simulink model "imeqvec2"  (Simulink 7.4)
settings: Solver=ode45  StartTime=0.0  StopTime=1  MaxStep=1e-3  RelTol=1e-3
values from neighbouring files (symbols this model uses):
  H = 0.60    (= 0.6)    [IMabc2.m]    (also in IMcur0.m = 0.3; imdef0vec.m = 0.3; imdef1vec.m = 0.3; imdef2vec.m = 0.3)
  ic = [fs0 fr0]    [imdef0vec.m]    (also in imdef1vec.m; imdef2vec.m = F; imic2.m = [phids phiqs phidr phiqr n0]'; imic3.m = [phids phiqs phidr phiqr n0]')
  Lm = eval(get(hLm,'String'))    [im3d.m]    (also in IMabc2.m = 4.5; imabcparam.m = 0.0847; IMabcrun0.m = 0.0847; IMabcrun1.m = 0.0847)
  Lrl = eval(get(hLr,'String'))    [im3d.m]    (also in IMabc2.m = 0.1; imabcparam.m = 0.0025; IMabcrun0.m = 0.0025; IMabcrun1.m = 0.0025)
  Lsl = eval(get(hLs,'String'))    [im3d.m]    (also in IMabc2.m = 0.1; imabcparam.m = 0.0025; IMabcrun0.m = 0.0025; IMabcrun1.m = 0.0025)
  n0 = 0.98    [imdef0vec.m]    (also in imdef1vec.m = 0.978; imdef2vec.m; imdefrotflux.m; imdefSIvec1.m = 0.95)
  Rr = input('Rotor resistance)[default = 2] =')    [Actac.m]    (also in im1phase.m = 0.3; im3d.m = eval(get(hRr,'String')); IMabc2.m = 0.02; imabcparam.m = 0.408)
  Rs = eval(get(hRs,'String'))    [im3d.m]    (also in IMabc2.m = 0.01; imabcparam.m = 0.531; IMabcrun0.m = 0.531; IMabcrun1.m = 0.531)
  Tl0 = Is*conj(Is)*Req    [imdef0vec.m]    (also in imdef1vec.m; imdef2vec.m = Lm*(I(2)*I(3)-I(1)*I(4)); imdefrotflux.m; imdefSIvec1.m = Te0/To)
  vs = 1.0    (= 1)    [imdef0vec.m]    (also in imdef1vec.m; imdef2vec.m; imdefrotflux.m; imdefSIvec1.m)
  wk = ws    (= 1)    [imdef0vec.m]    (also in imdef1vec.m; imdef2vec.m; imdefrotflux.m; imdefSIvec1.m)
  wo = 2*pi*freq0    [calc0.m]    (also in IMabc2.m = 376.991118431; imabcparam.m = 376.991118431; IMabcrun0.m = 376.991118431; IMabcrun1.m = 376.991118431)

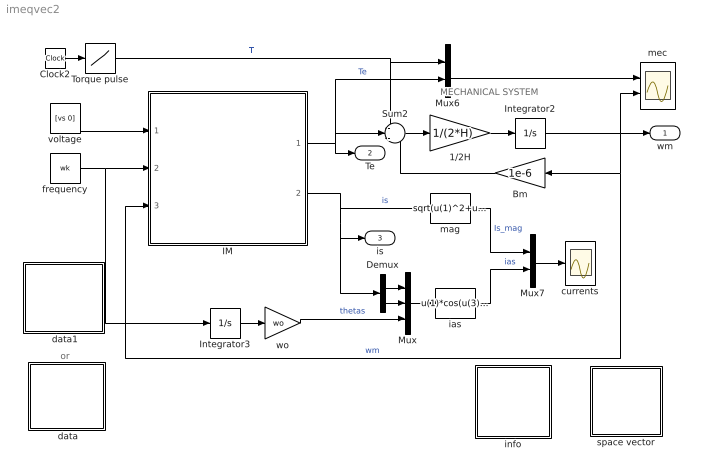
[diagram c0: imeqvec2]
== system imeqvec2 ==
  note: or
  note: MECHANICAL SYSTEM
  " data" : Subsystem
  " data1" : Subsystem
  1/2H : Gain  Gain=1/(2*H)  ParameterDataType=sfix(16)  ParameterScaling=2^0  OutDataType=sfix(16)  OutScaling=2^0
  Bm : Gain  Gain=1e-6  ParameterDataType=sfix(16)  ParameterScaling=2^0  OutDataType=sfix(16)  OutScaling=2^0
  Clock2 : Clock
  Demux : Demux  Outputs=2
  IM : Subsystem
  Integrator2 : Integrator  InitialCondition=n0
  Integrator3 : Integrator
  Mux : Mux  Inputs=3
  Mux6 : Mux  Inputs=2
  Mux7 : Mux  Inputs=2
  Sum2 : Sum  Inputs=-+-  OutDataType=sfix(16)  OutScaling=2^0
  Torque pulse : Lookup  InputValues=[0 0.1 0.1 0.5 0.5 2]  Table="[Tl0 Tl0  0 0 0.5 0.5]"  OutDataType=sfix(16)  OutScaling=2^0
  currents : Scope
  frequency : Constant  Value=wk  OutDataType=sfix(16)  OutScaling=2^0
  ias : Fcn  Expr=u(1)*cos(u(3))-u(2)*sin(u(3))
  info : Subsystem
  mag : Fcn  Expr=sqrt(u(1)^2+u(2)^2)
  mec : Scope  NumInputPorts=2
  space vector : Subsystem
  voltage : Constant  Value=[vs 0]  OutDataType=sfix(16)  OutScaling=2^0
  wo : Gain  Gain=wo  ParameterDataType=sfix(16)  ParameterScaling=2^0  OutDataType=sfix(16)  OutScaling=2^0
  wm : Outport
  Te : Outport  Port=2
  is : Outport  Port=3
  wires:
  voltage/1 -> IM/1(vs)
  frequency/1 -> Integrator3/1, IM/2(wk)
  Demux/1 -> Mux/1
  Demux/2 -> Mux/2
  Mux/1 -> ias/1
  ias/1 -> Mux7/2  "ias"
  mag/1 -> Mux7/1  "Is_mag"
  Mux7/1 -> currents/1
  IM/2(is) -> mag/1, Demux/1, is/1  "is"
  Sum2/1 -> 1/2H/1
  1/2H/1 -> Integrator2/1
  Mux6/1 -> mec/1
  IM/1(Te) -> Sum2/2, Mux6/2, Te/1  "Te"
  Bm/1 -> Sum2/3
  Integrator3/1 -> wo/1
  wo/1 -> Mux/3  "thetas"
  Integrator2/1 -> mec/2, wm/1, IM/3(wm), Bm/1  "wm"
  Clock2/1 -> Torque pulse/1
  Torque pulse/1 -> Mux6/1, Sum2/1  "Tl"

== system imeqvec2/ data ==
  note: This demo simulates the running of an induction motor in steady-state when a sudden input change is effected: a)torque step changes at constant voltage excitation b) voltage input sag at constant frequency and load torque c)simultaneous step changes in voltage magnitude and frequency
  note: Double click the block to enter the machine parameters and initial conditions and then run the simulation

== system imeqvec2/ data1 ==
  note: This demo simulates the running of an induction motor in steady-state when a sudden input change is effected: a)torque step changes at constant voltage excitation b) voltage input sag at constant frequency and load torque c)simultaneous step changes in voltage magnitude and frequency
  note: Double click the block to enter the machine parameters and initial conditions and then run the simulation

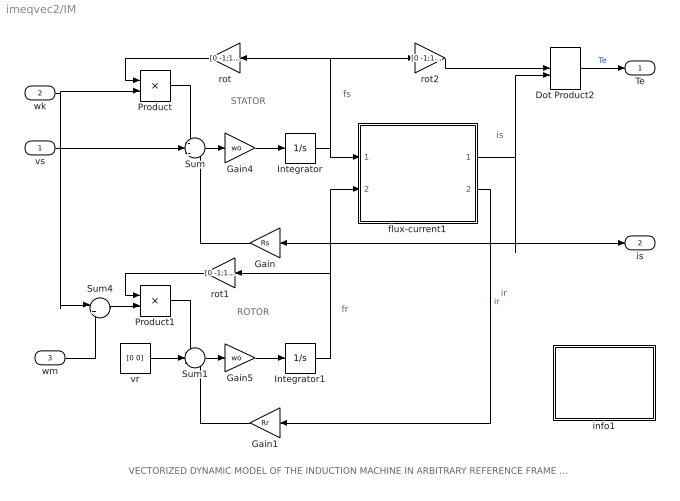
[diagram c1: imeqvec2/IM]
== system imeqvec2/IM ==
  note: ROTOR
  note: STATOR
  note: fs
  note: fr
  note: is
  note: VECTORIZED DYNAMIC MODEL OF THE INDUCTION MACHINE IN ARBITRARY REFERENCE FRAME (per unit formulation)
  note: ir
  vs : Inport  OutDataType=sfix(16)  OutScaling=2^0
  wk : Inport  Port=2  OutDataType=sfix(16)  OutScaling=2^0
  wm : Inport  Port=3  OutDataType=sfix(16)  OutScaling=2^0
  Dot Product2 : DotProduct  OutDataType=fixdt(1, 16)  OutScaling=2^-10
  Gain : Gain  Gain=Rs  ParameterDataType=sfix(16)  ParameterScaling=2^0  OutDataType=sfix(16)  OutScaling=2^0
  Gain1 : Gain  Gain=Rr  ParameterDataType=sfix(16)  ParameterScaling=2^0  OutDataType=sfix(16)  OutScaling=2^0
  Gain4 : Gain  Gain=wo  ParameterDataType=sfix(16)  ParameterScaling=2^0  OutDataType=sfix(16)  OutScaling=2^0
  Gain5 : Gain  Gain=wo  ParameterDataType=sfix(16)  ParameterScaling=2^0  OutDataType=sfix(16)  OutScaling=2^0
  Integrator : Integrator  InitialCondition=[ic(1) ic(2)]
  Integrator1 : Integrator  InitialCondition=[ic(3) ic(4)]
  Product : Product  OutDataType=sfix(16)  OutScaling=2^0
  Product1 : Product  OutDataType=sfix(16)  OutScaling=2^0
  Sum : Sum  Inputs=-+-  OutDataType=sfix(16)  OutScaling=2^0
  Sum1 : Sum  Inputs=-+-  OutDataType=sfix(16)  OutScaling=2^0
  Sum4 : Sum  Inputs=|+-  OutDataType=sfix(16)  OutScaling=2^0
  flux-current1 : Subsystem
  info1 : Subsystem  AncestorBlock=mrlib/IM/info
  rot : Gain  Gain=[0 -1;1 0]  Multiplication=Matrix(K*u)  ParameterDataType=sfix(16)  ParameterScaling=2^0  OutDataType=sfix(16)  OutScaling=2^0
  rot1 : Gain  Gain=[0 -1;1 0]  Multiplication=Matrix(K*u)  ParameterDataType=sfix(16)  ParameterScaling=2^0  OutDataType=sfix(16)  OutScaling=2^0
  rot2 : Gain  Gain=[0 -1;1 0]  Multiplication=Matrix(K*u)  ParameterDataType=sfix(16)  ParameterScaling=2^0  OutDataType=sfix(16)  OutScaling=2^0
  vr : Constant  Value=[0 0]  OutDataType=sfix(16)  OutScaling=2^0
  Te : Outport
  is : Outport  Port=2
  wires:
  Gain/1 -> Sum/3
  vr/1 -> Sum1/2
  Gain1/1 -> Sum1/3
  flux-current1/2(ir) -> Gain1/1  "ir"
  Integrator/1 -> flux-current1/1(fs), rot/1, rot2/1
  Integrator1/1 -> rot1/1, flux-current1/2(fr)
  Product1/1 -> Sum1/1
  rot1/1 -> Product1/1
  Product/1 -> Sum/1
  rot/1 -> Product/1
  rot2/1 -> Dot Product2/1
  Sum4/1 -> Product1/2
  Sum/1 -> Gain4/1
  Gain4/1 -> Integrator/1
  Sum1/1 -> Gain5/1
  Gain5/1 -> Integrator1/1
  flux-current1/1(is) -> Gain/1, is/1, Dot Product2/2
  Dot Product2/1 -> Te/1  "Te"
  vs/1 -> Sum/2
  wk/1 -> Product/2, Sum4/1
  wm/1 -> Sum4/2

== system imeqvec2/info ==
  note: The induction machine is modeled in vectorized form in conformity with the space vector formulation. This one-to-one correspondence can be seen by clicking both the INDUCTION MACHINE subsystem block and the MATHEMATICAL MODEL equation block. The synchronous reference frame is chosen here because the machine is operating under balanced three-phase sinusoidal excitation; the input voltage is thefore constant as indicated. The parameters describing the electromechanical system are expressed in per unit and are entered after double-clicking one of the PARAMETERS/IC blocks. The system is initially assumed to be operated under load in a steady state defined by a specified speed. The initial conditions are established by calling a phasor calculation based on the standard steady-state equivalent circuit of the induction machine. The simulation can then be run. In the present case, it exhibits the dynamic response to a pulsed applied torque. The torque developed, the speed, and the stator current are observed on the scopes . The torque-speed dynamic characteristics can then be obtained after double clicking the X-Y PLOT block.
  note: Running of a Line-Fed Induction Motor Synchronous frame Per unit system

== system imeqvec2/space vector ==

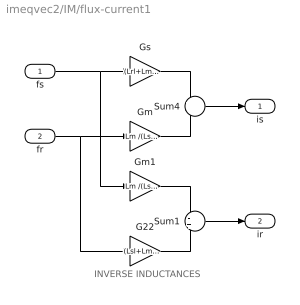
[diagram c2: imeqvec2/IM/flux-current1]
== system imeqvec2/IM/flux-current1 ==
  note: INVERSE INDUCTANCES
  fs : Inport  OutDataType=sfix(16)  OutScaling=2^0
  fr : Inport  Port=2  OutDataType=sfix(16)  OutScaling=2^0
  G22 : Gain  Gain=(Lsl+Lm )/(Lsl*Lrl+Lsl*Lm+Lrl*Lm)  ParameterDataType=sfix(16)  ParameterScaling=2^0  OutDataType=sfix(16)  OutScaling=2^0
  Gm : Gain  Gain=Lm /(Lsl*Lrl+Lsl*Lm+Lrl*Lm)  ParameterDataType=sfix(16)  ParameterScaling=2^0  OutDataType=sfix(16)  OutScaling=2^0
  Gm1 : Gain  Gain=Lm /(Lsl*Lrl+Lsl*Lm+Lrl*Lm)  ParameterDataType=sfix(16)  ParameterScaling=2^0  OutDataType=sfix(16)  OutScaling=2^0
  Gs : Gain  Gain=(Lrl+Lm) /(Lsl*Lrl+Lsl*Lm+Lrl*Lm)  ParameterDataType=sfix(16)  ParameterScaling=2^0  OutDataType=sfix(16)  OutScaling=2^0
  Sum1 : Sum  Inputs=-+  OutDataType=sfix(16)  OutScaling=2^0
  Sum4 : Sum  Inputs=+-  OutDataType=sfix(16)  OutScaling=2^0
  is : Outport
  ir : Outport  Port=2
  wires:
  fs/1 -> Gs/1, Gm1/1
  Gs/1 -> Sum4/1
  fr/1 -> Gm/1, G22/1
  Gm/1 -> Sum4/2
  Sum4/1 -> is/1
  Gm1/1 -> Sum1/1
  G22/1 -> Sum1/2
  Sum1/1 -> ir/1

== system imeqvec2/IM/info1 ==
  note: Electrical system equations: vs = Rs is + 1/wo (dfs/dt) + wk M(pi/2) fs vr = Rr ir + 1/wo (dfr/dt) + (wk - wm) M(pi/2) fr where the variables i, v, and f are 2-dimensional space vectors; for instance is = [ids iqs] and so forth, wk is the speed of the reference frame, wm the rotor speed, and M(pi/2)represents a 90o space rotator namely M(pi/2) = [0 -1;1 0] The flux linkage current relations are: fs = Ls is + Lm ir or is = Gs fs - Gm Fr fr = Lm is + Lr ir ir = -Gm fs + Gr fr where Ls =Lm +Lsl and Lr = Lm +Lrl Gs = Lr / delta ; Gm = Lm / delta ; Gr= Ls / delta delta = Lsl*Lrl + Lm*Lsl + Lm* Lrl Mechanical system equations: Te = 2H (dwm/dt ) + Bm wm + Tl where Te = fs (cross) is = M(pi/2) fs (dot) is = fds iqs - fqs ids = fs x is = M(pi/2) fs . is = ir x fr = Lm (ir x is) = Lm/Lr (fr x is) = Gm (fr x fs)
  note: Mathematical model of the induction machine. Space vector formulation in an arbitrary dq common reference frame. Per unit description.
